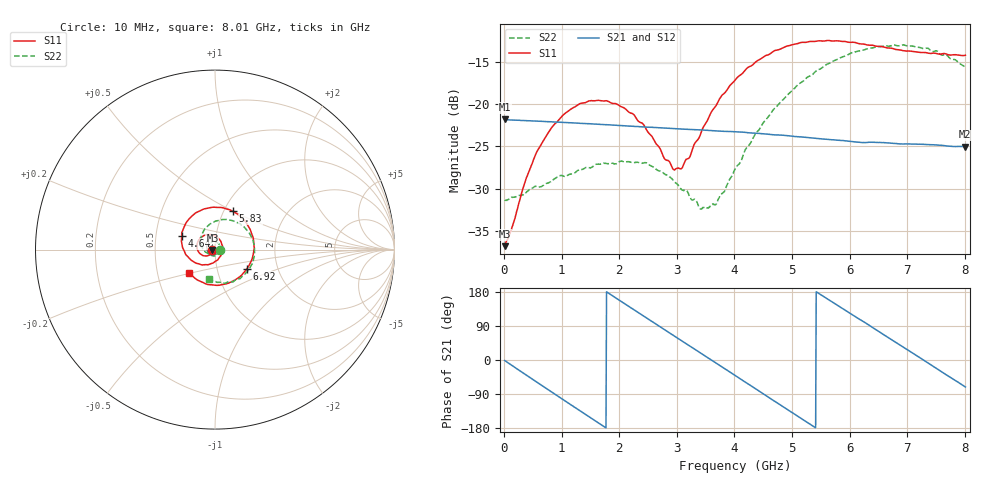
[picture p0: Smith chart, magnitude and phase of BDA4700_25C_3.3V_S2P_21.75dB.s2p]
!Agilent Technologies,E5071B,MY42404982,A.09.10
!Date: Mon Oct 20 18:12:11 2025
!Data & Calibration Information:
!Freq	S11:SOLT2(ON)	S21:SOLT2(ON)	S12:SOLT2(ON)	S22:SOLT2(ON)
# Hz S RI R 50
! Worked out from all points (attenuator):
!   801 points, 10 MHz to 8.01 GHz, reference 50 ohm
!   highest |S21| = -21.82 dB at 10 MHz (marker M1); lowest = -25.0 dB at 8 GHz (marker M2)
!   lowest |S11| = -36.8 dB at 10 MHz (marker M3), VSWR 1.03, Z = 48.6 - j0.129 ohm
!   |S11| at or under -10 dB: start of sweep to end of sweep
!   |S22| runs from -32.4 to -13.0 dB; largest |S21 - S12| = 0.00096
!   S11 on the Smith chart (normalised r, x): 10 MHz: 0.97, -0.00; 4.64 GHz: 0.68, +0.11; 5.83 GHz: 1.11, +0.50; 6.92 GHz: 1.39, -0.31; 8.01 GHz: 0.73, -0.20
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1e7  -0.0144 -0.00133  0.0811 -0.00176  0.081 -0.00182  0.027 -0.000781
5.9e8  -0.0409 -0.035  0.039 -0.0689  0.039 -0.0689  0.0139 -0.0294
1.01e9  -0.0816 -0.0243  -0.0174 -0.0759  -0.0173 -0.076  -0.0153 -0.0346
1.35e9  -0.1008 0.0101  -0.0563 -0.0523  -0.0563 -0.0524  -0.0368 -0.0182
1.77e9  -0.0836 0.0629  -0.0755 -0.00108  -0.0755 -0.00107  -0.0427 0.0129
2.08e9  -0.0453 0.0836  -0.0644 0.0374  -0.0645 0.0374  -0.0299 0.0343
2.68e9  0.0327 0.0457  -0.000562 0.0724  -0.000674 0.0724  0.0136 0.038
2.94e9  0.0408 0.00454  0.0304 0.0647  0.0303 0.0646  0.0259 0.0241
3.08e9  0.0368 -0.0192  0.0449 0.0552  0.0443 0.0555  0.0285 0.0129
3.41e9  0.000262 -0.066  0.0666 0.0225  0.0667 0.0225  0.0209 -0.0117
3.54e9  -0.0219 -0.0782  0.0695 0.00706  0.0696 0.00701  0.0137 -0.0202
3.69e9  -0.0525 -0.084  0.0685 -0.0108  0.0686 -0.011  0.00104 -0.0258
4.01e9  -0.1211 -0.0664  0.0521 -0.0447  0.0522 -0.0445  -0.0317 -0.0261
4.64e9  -0.1854 0.076  -0.015 -0.0643  -0.0148 -0.0643  -0.0788 0.0408
5.35e9  -0.0535 0.2281  -0.0626 -0.00764  -0.0626 -0.008  -0.0156 0.148
5.83e9  0.1008 0.2129  -0.047 0.039  -0.0468 0.039  0.0918 0.1629
6.25e9  0.1967 0.1109  -0.0107 0.0582  -0.00976 0.0583  0.1806 0.105
6.68e9  0.2113 -0.0344  0.031 0.0501  0.0312 0.05  0.2195 -0.00127
6.92e9  0.1763 -0.1081  0.0474 0.0334  0.0475 0.0332  0.2124 -0.0685
7.47e9  0.0162 -0.1991  0.0544 -0.0183  0.0544 -0.0184  0.1059 -0.1755
8e9  -0.1417 -0.132  0.0189 -0.0528  0.019 -0.0528  -0.0291 -0.1632
8.01e9  -0.1439 -0.1302  0.018 -0.0531  0.0181 -0.053  -0.0315 -0.1616
